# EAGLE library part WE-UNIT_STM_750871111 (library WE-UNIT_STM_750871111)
Off-Line Transformer WE-Unit STM - Nominal input voltage: 85-265 VAC - Operating temperature: -40°C to +125 °C - Isolation voltage 4 kVAC -- Especially designed for several ICs from STMicroelectronics VIPer 27L -- Universal input -- Offline-switch mode power supplies
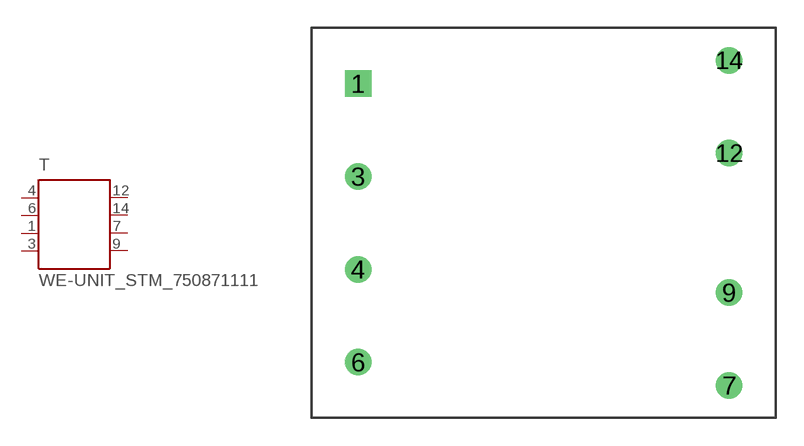
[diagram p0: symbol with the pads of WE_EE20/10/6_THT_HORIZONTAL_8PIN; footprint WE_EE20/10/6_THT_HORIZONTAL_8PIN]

Designator prefix T

## WE-UNIT_STM_750871111 (MPN: 750871111; OC_FARNELL: 1849051; OC_NEWARK: 13T9844; PACKAGE: EE20/10/6_THT_HORIZONTAL_8PIN; SUPPLIER: Würth Elektronik eiSos GmbH)  [WE_EE20/10/6_THT_HORIZONTAL_8PIN]
1  2  pas
3  1  pas
4  4  pas
6  3  pas
7  7  pas
9  8  pas
12  5  pas
14  6  pas

## Footprint WE_EE20/10/6_THT_HORIZONTAL_8PIN (pad centres in mm)
Transformer, EE20/10/6 THT Horizontal 8 Pin
drill 0.92 square: 1 -10,7.5
drill 0.92: 3 -10,2.5; 4 -10,-2.5; 6 -10,-7.5; 7 10,-8.75; 9 10,-3.75; 12 10,3.75; 14 10,8.75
